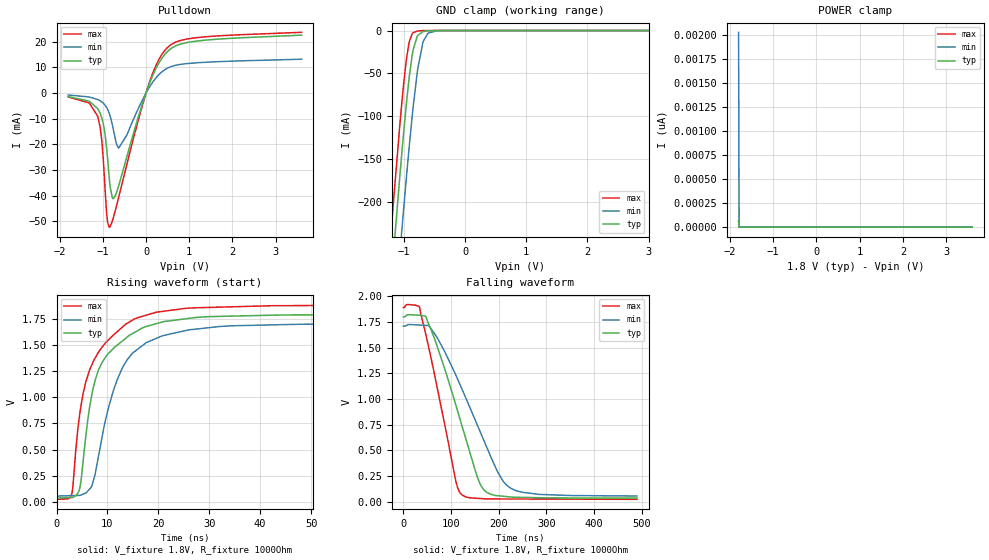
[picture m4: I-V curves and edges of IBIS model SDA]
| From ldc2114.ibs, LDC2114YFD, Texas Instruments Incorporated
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|   Model SDA
[Model]   SDA
Model_type   I/O_open_drain
Polarity   Non-Inverting
Enable   Active-Low
Vinl = .513
Vinh = 1.323
Vmeas = 0.9
Vref = 1.8
Cref = 15pF
Rref = 1000
|   typ   min   max
|   (nom PVT)   (slow PVT)   (fast PVT)
C_comp   1.077p   1.038p   1.123p
|C_comp (ON state)   1.077p   1.038p   1.123p
|C_comp (OFF state)   1.167p   .   1.134p   1.226p
[Voltage Range]   1.8   1.71   1.89
[Temperature Range]   27   125   -40
[Pullup Reference]   1.8   1.71   1.89
[Pulldown Reference]   0   0   0
[Power Clamp Reference]   1.8   1.71   1.89
[GND Clamp Reference]   0   0   0
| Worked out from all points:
|   slope of the pulldown table from 0 to 0.27 V, typ, clamps not added: 24.9 ohm
|   GND clamp passes 1 mA (typ) near -0.67 V on its own axis
|   falling waveform, V_fixture 1.8V, R_fixture 1000Ohm: 20-80 % time 69.7ns typ, 93.2ns min, 49.3ns max; typ from 1.8 V to 0.035 V
|   rising waveform, V_fixture 1.8V, R_fixture 1000Ohm: 20-80 % time 5.52ns typ, 6.13ns min, 5.89ns max; typ from 0.035 V to 1.8 V
[Pulldown]
|   Voltage   I(typ)   I(min)   I(max)
-1.8V     -1.393mA   -749.2uA   -1.527mA
-1.33V    -3.082mA   -1.495mA   -3.761mA
-1.12V    -5.994mA   -2.483mA   -8.967mA
-1.028V   -9.403mA   -3.364mA   -17.75mA
-968.4mV  -13.79mA   -4.272mA   -31.36mA
-909mV    -21.78mA   -5.667mA   -47.16mA
-844.2mV  -34.15mA   -8.169mA   -52.21mA
-768.6mV  -41.1mA    -13.16mA   -49.24mA
-633.6mV  -36.24mA   -21.45mA   -40.64mA
46.8mV    2.243mA    1.406mA    2.544mA
478.8mV   15.88mA    9.542mA    17.44mA
3.6V      22.55mA    13.18mA    23.65mA
[GND Clamp]
|   Voltage   I(typ)   I(min)   I(max)
-1.8V     -850.8mA   -939.7mA   -793.3mA
-1.206V   -290.8mA   -383.1mA   -229.8mA
-1.19V    -276.2mA   -368.6mA   -215.3mA
-1.066V   -168.1mA   -259.2mA   -108.4mA
-1.033V   -141.4mA   -231.6mA   -82.96mA
-968.4mV  -91.21mA   -178mA     -38.56mA
-919.8mV  -58.08mA   -139.7mA   -15.54mA
-849.6mV  -22.44mA   -89.12mA   -2.553mA
-774mV    -5.691mA   -44.51mA   -541.9uA
-693mV    -1.419mA   -14.75mA   -88.58uA
-606.6mV  -268.9uA   -3.019mA   -5.932uA
3.6V      0A         0A         0A
[POWER Clamp]
|   Voltage   I(typ)   I(min)   I(max)
-1.8V     66.46pA    2.024nA    63.65pA
-1.789V   0A         0A         0A
-1.784V   0A         0A         0A
3.6V      0A         0A         0A
[Ramp]
R_load = 1000
|   typ   min   max
dV/dt_r   1.05911/5.45645e-09   0.993678/6.09376e-09   1.1204/5.89747e-09
dV/dt_f   1.05906/6.95037e-08   0.993121/9.28817e-08   1.1204/4.92764e-08
[Falling Waveform]
V_fixture = 1.8V
V_fixture_min = 1.71V
V_fixture_max = 1.89V
R_fixture = 1000Ohm
C_fixture = 0F
|   Time   V(typ)   V(min)   V(max)
0s        1.8V       1.71V      1.89V
33.92ns   1.815V     1.719V     1.892V
47.56ns   1.799V     1.716V     1.617V
58.56ns   1.67V      1.679V     1.385V
109.7ns   945.9mV    1.235V     208.6mV
123ns     738.1mV    1.095V     65.34mV
168ns     120.2mV    606mV      28.67mV
198.4ns   57.39mV    284.2mV    26.32mV
224.5ns   45.96mV    133.5mV    25.99mV
490ns     34.91mV    54.8mV     22.66mV
[Rising Waveform]
V_fixture = 1.8V
V_fixture_min = 1.71V
V_fixture_max = 1.89V
R_fixture = 1000Ohm
C_fixture = 0F
|   Time   V(typ)   V(min)   V(max)
0s        34.81mV    53.86mV    22.66mV
2.947ns   39.85mV    57.96mV    67.56mV
4.432ns   106.5mV    60.03mV    792.8mV
6.522ns   913.7mV    122mV      1.265V
8.398ns   1.278V     476.2mV    1.445V
11.04ns   1.462V     1.044V     1.592V
13.84ns   1.576V     1.358V     1.709V
17.64ns   1.68V      1.525V     1.788V
25.22ns   1.752V     1.639V     1.852V
490ns     1.8V       1.71V      1.89V
